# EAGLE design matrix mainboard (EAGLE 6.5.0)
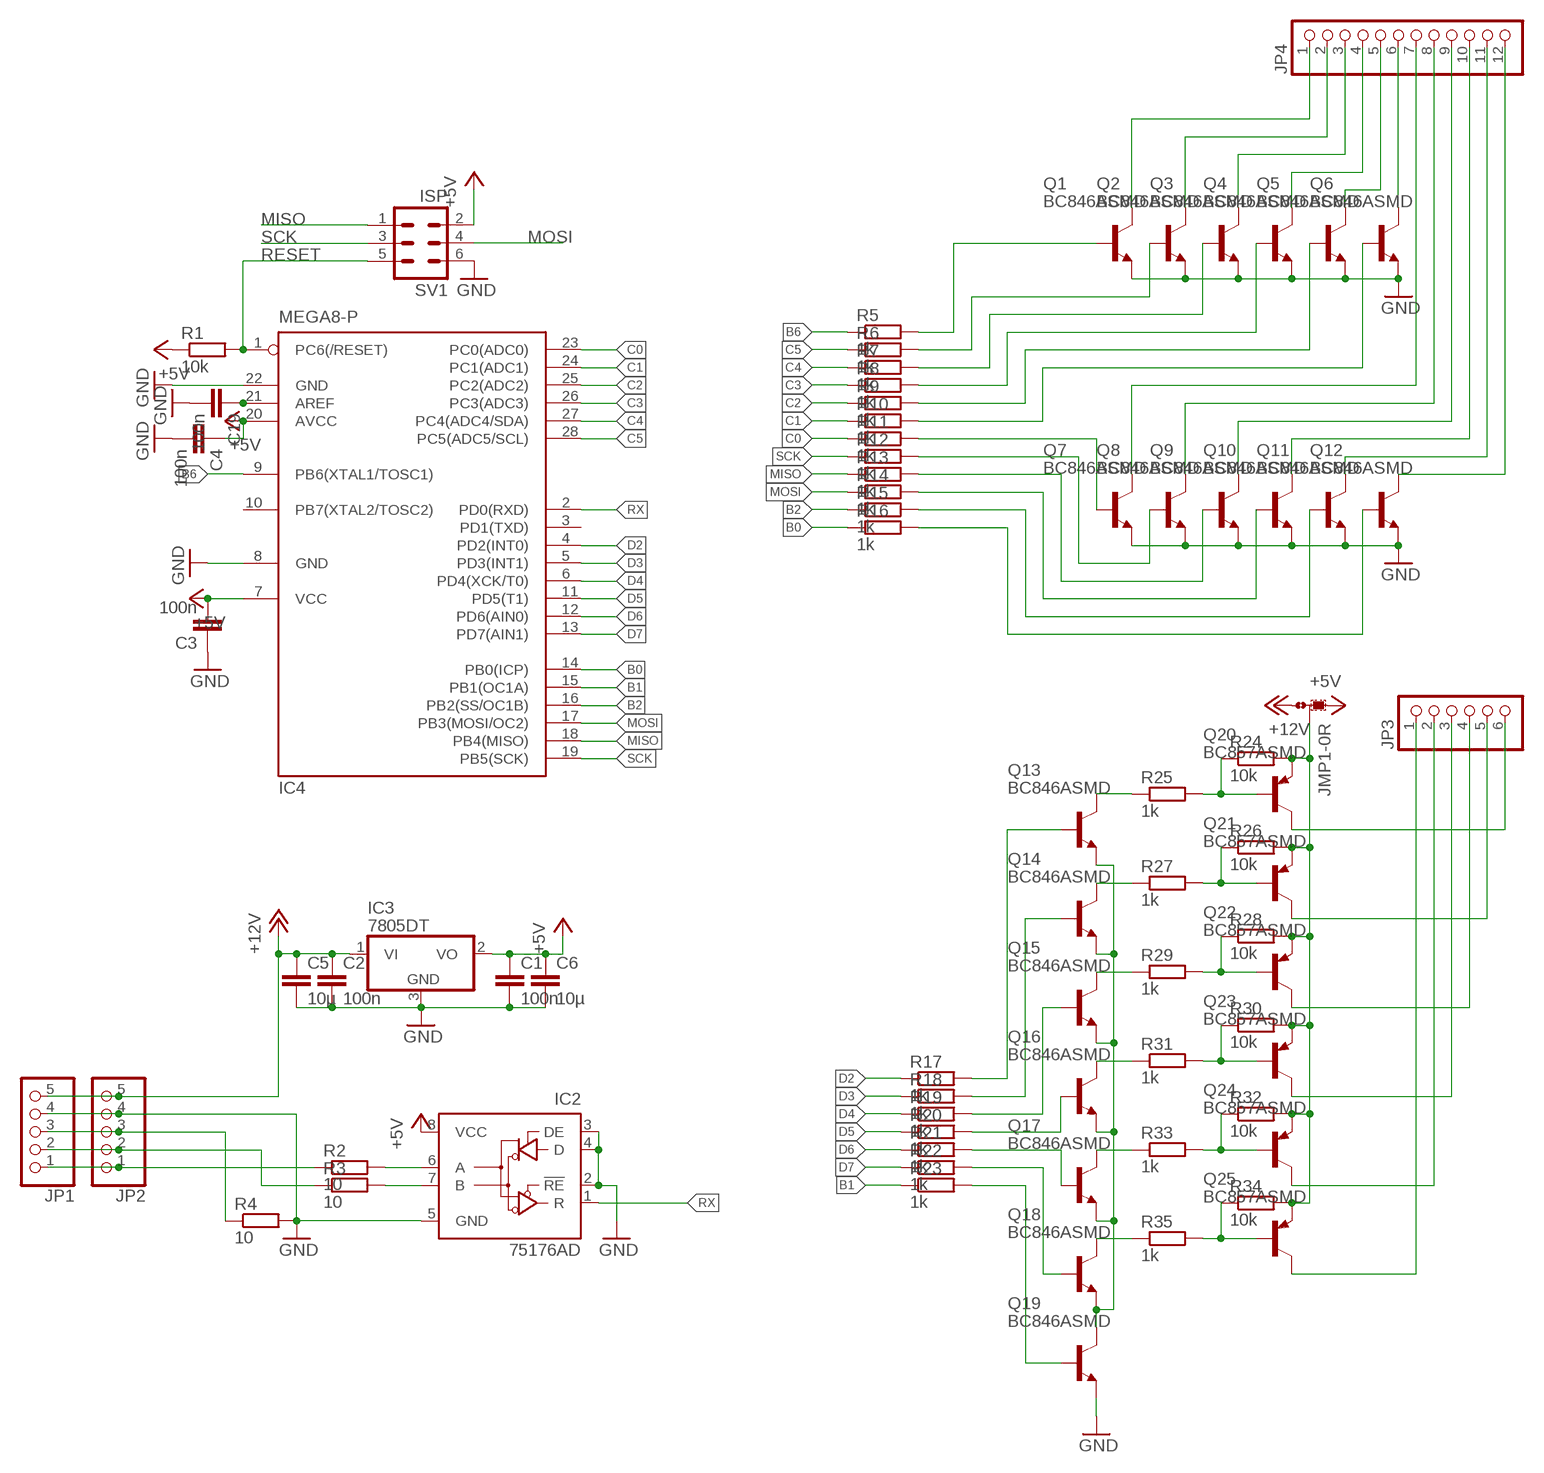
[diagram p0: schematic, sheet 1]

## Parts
C1  100n  C-EUC0805K  [C0805K]
C2  100n  C-EUC0805K  [C0805K]
C3  100n  C-EUC0805K  [C0805K]
C4  100n  C-EUC0805K  [C0805K]
C5  10µ  C-EUC0805K  [C0805K]
C6  10µ  C-EUC0805K  [C0805K]
C19  100n  C-EUC0805K  [C0805K]
IC2  75176AD  [D_R-PDSO-G8]
IC3  7805DT  [TO252]
IC4  MEGA8-P  [DIL28-3]
JMP1  0R-JUMPA  [A0R-JMP]
JP1  PINHD-1X5  [1X05]
JP2  PINHD-1X5  [1X05]
JP3  PINHD-1X6  [1X06]
JP4  PINHD-1X12  [1X12]
Q1  BC846ASMD  [SOT23]
Q2  BC846ASMD  [SOT23]
Q3  BC846ASMD  [SOT23]
Q4  BC846ASMD  [SOT23]
Q5  BC846ASMD  [SOT23]
Q6  BC846ASMD  [SOT23]
Q7  BC846ASMD  [SOT23]
Q8  BC846ASMD  [SOT23]
Q9  BC846ASMD  [SOT23]
Q10  BC846ASMD  [SOT23]
Q11  BC846ASMD  [SOT23]
Q12  BC846ASMD  [SOT23]
Q13  BC846ASMD  [SOT23]
Q14  BC846ASMD  [SOT23]
Q15  BC846ASMD  [SOT23]
Q16  BC846ASMD  [SOT23]
Q17  BC846ASMD  [SOT23]
Q18  BC846ASMD  [SOT23]
Q19  BC846ASMD  [SOT23]
Q20  BC857ASMD  [SOT23-BEC]
Q21  BC857ASMD  [SOT23-BEC]
Q22  BC857ASMD  [SOT23-BEC]
Q23  BC857ASMD  [SOT23-BEC]
Q24  BC857ASMD  [SOT23-BEC]
Q25  BC857ASMD  [SOT23-BEC]
R1  10k  R-EU_M0805  [M0805]
R2  10  R-EU_M0805  [M0805]
R3  10  R-EU_M0805  [M0805]
R4  10  R-EU_M0805  [M0805]
R5  1k  R-EU_M0805  [M0805]
R6  1k  R-EU_M0805  [M0805]
R7  1k  R-EU_M0805  [M0805]
R8  1k  R-EU_M0805  [M0805]
R9  1k  R-EU_M0805  [M0805]
R10  1k  R-EU_M0805  [M0805]
R11  1k  R-EU_M0805  [M0805]
R12  1k  R-EU_M0805  [M0805]
R13  1k  R-EU_M0805  [M0805]
R14  1k  R-EU_M0805  [M0805]
R15  1k  R-EU_M0805  [M0805]
R16  1k  R-EU_M0805  [M0805]
R17  1k  R-EU_M0805  [M0805]
R18  1k  R-EU_M0805  [M0805]
R19  1k  R-EU_M0805  [M0805]
R20  1k  R-EU_M0805  [M0805]
R21  1k  R-EU_M0805  [M0805]
R22  1k  R-EU_M0805  [M0805]
R23  1k  R-EU_M0805  [M0805]
R24  10k  R-EU_M0805  [M0805]
R25  1k  R-EU_M0805  [M0805]
R26  10k  R-EU_M0805  [M0805]
R27  1k  R-EU_M0805  [M0805]
R28  10k  R-EU_M0805  [M0805]
R29  1k  R-EU_M0805  [M0805]
R30  10k  R-EU_M0805  [M0805]
R31  1k  R-EU_M0805  [M0805]
R32  10k  R-EU_M0805  [M0805]
R33  1k  R-EU_M0805  [M0805]
R34  10k  R-EU_M0805  [M0805]
R35  1k  R-EU_M0805  [M0805]
SV1  ISP  ML6  [ML6]

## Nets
+5V: C1.1 C3.2 C4.1 C6.1 IC2.8(VCC) IC3.2(VO) IC4.7(VCC) IC4.20(AVCC) JMP1.1 R1.1 SV1.2
+12V: C2.1 C5.1 IC3.1(VI) JMP1.3 JP1.5 JP2.5
B0: IC4.14(PB0(ICP)) R16.1
B1: IC4.15(PB1(OC1A)) R23.1
B2: IC4.16(PB2(SS/OC1B)) R15.1
B6: IC4.9(PB6(XTAL1/TOSC1)) R5.1
C0: IC4.23(PC0(ADC0)) R11.1
C1: IC4.24(PC1(ADC1)) R10.1
C2: IC4.25(PC2(ADC2)) R9.1
C3: IC4.26(PC3(ADC3)) R8.1
C4: IC4.27(PC4(ADC4/SDA)) R7.1
C5: IC4.28(PC5(ADC5/SCL)) R6.1
D2: IC4.4(PD2(INT0)) R17.1
D3: IC4.5(PD3(INT1)) R18.1
D4: IC4.6(PD4(XCK/T0)) R19.1
D5: IC4.11(PD5(T1)) R20.1
D6: IC4.12(PD6(AIN0)) R21.1
D7: IC4.13(PD7(AIN1)) R22.1
GND: C1.2 C2.2 C3.1 C4.2 C5.2 C6.2 C19.2 IC2.2(!RE) IC2.3(DE) IC2.4(D) IC2.5(GND) IC3.3(GND) IC4.8(GND) IC4.22(GND) JP1.4 JP2.4 Q1.2(E) Q2.2(E) Q3.2(E) Q4.2(E) Q5.2(E) Q6.2(E) Q7.2(E) Q8.2(E) Q9.2(E) Q10.2(E) Q11.2(E) Q12.2(E) Q19.2(E) R4.2 SV1.6
MISO: IC4.18(PB4(MISO)) R13.1 SV1.1
MOSI: IC4.17(PB3(MOSI/OC2)) R14.1 SV1.4
N$1: JP1.1 JP2.1 R2.1
N$2: JP1.2 JP2.2 R3.1
N$3: JP1.3 JP2.3 R4.1
N$4: Q1.1(B) R5.2
N$6: IC2.6(A) R2.2
N$7: IC2.7(B) R3.2
N$8: Q2.1(B) R6.2
N$9: Q13.1(B) R17.2
N$10: Q14.1(B) R18.2
N$11: Q3.1(B) R7.2
N$12: Q4.1(B) R8.2
N$13: Q5.1(B) R9.2
N$14: Q6.1(B) R10.2
N$15: JP4.6 Q6.3(C)
N$16: JP4.5 Q5.3(C)
N$17: JP4.4 Q4.3(C)
N$18: JP4.3 Q3.3(C)
N$19: JP4.2 Q2.3(C)
N$20: JP4.1 Q1.3(C)
N$21: JP4.7 Q7.3(C)
N$22: JP4.8 Q8.3(C)
N$23: JP4.9 Q9.3(C)
N$24: JP4.10 Q10.3(C)
N$25: JP4.11 Q11.3(C)
N$26: JP4.12 Q12.3(C)
N$27: Q7.1(B) R11.2
N$28: Q8.1(B) R12.2
N$29: C19.1 IC4.21(AREF)
N$30: Q9.1(B) R13.2
N$31: Q10.1(B) R14.2
N$32: Q11.1(B) R15.2
N$33: Q12.1(B) R16.2
N$34: Q15.1(B) R19.2
N$35: Q16.1(B) R20.2
N$36: Q17.1(B) R21.2
N$37: Q18.1(B) R22.2
N$38: JMP1.2 Q20.E Q21.E Q22.E Q23.E Q24.E Q25.E R24.2 R26.2 R28.2 R30.2 R32.2 R34.2
N$39: Q21.B R26.1 R27.2
N$40: Q13.2(E) Q14.2(E) Q15.2(E) Q16.2(E) Q17.2(E) Q18.2(E) Q19.3(C)
N$41: Q19.1(B) R23.2
N$43: Q22.B R28.1 R29.2
N$44: Q23.B R30.1 R31.2
N$51: Q24.B R32.1 R33.2
N$52: Q25.B R34.1 R35.2
N$53: Q20.B R24.1 R25.2
N$54: Q13.3(C) R25.1
N$55: Q14.3(C) R27.1
N$56: Q15.3(C) R29.1
N$57: Q16.3(C) R31.1
N$58: Q17.3(C) R33.1
N$59: Q18.3(C) R35.1
N$60: JP3.6 Q20.C
N$61: JP3.5 Q21.C
N$62: JP3.4 Q22.C
N$63: JP3.3 Q23.C
N$64: JP3.2 Q24.C
N$65: JP3.1 Q25.C
RESET: IC4.1(PC6(/RESET)) R1.2 SV1.5
RX: IC2.1(R) IC4.2(PD0(RXD))
SCK: IC4.19(PB5(SCK)) R12.1 SV1.3
Unconnected: IC4.3(PD1(TXD)) IC4.10(PB7(XTAL2/TOSC2))

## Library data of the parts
C1-C6 C19 = rcl:C-EU: CAPACITOR, European symbol
IC2 = 751xx:75176A: DIFFERENTIAL BUS TRANSCEIVER Source: http://focus.ti.com/lit/ds/symlink/sn75176a.pdf
IC3 = linear:78*: Positive VOLTAGE REGULATOR Source: http://cache.national.com/ds/LM/LM78L05.pdf http://www.fairchildsemi.com/ds/LM/LM7805.pdf
IC4 = atmel:MEGA8-P: MICROCONTROLLER 8 Kbytes FLASH, 1 kbytes SRAM, 512 bytes EEPROM, USART, 4-channel 10 bit ADC, 2-channel 8 bit ADC Pin compatible with Atmega48, ATMega88, ATMega168 Source: avr.lbr; OC_FARNELL: unknown; OC_NEWARK: unknown
JMP1 = jump-0r-smd:0R-JUMP: SMD 0R 0805 Jumper
JP1 JP2 = pinhead:PINHD-1X5: PIN HEADER
JP3 = pinhead:PINHD-1X6: PIN HEADER
JP4 = pinhead:PINHD-1X12: PIN HEADER
Q1-Q19 = transistor-npn:BC846*: NPN Transistor
Q20-Q25 = transistor-pnp:BC857*: PNP Transistror
R1-R35 = rcl:R-EU_: RESISTOR, European symbol
SV1 = con-harting-ml:ML6: HARTING

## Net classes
0 default: width 0.4 mm, drill 0.001 mm, clearance 0.25 mm

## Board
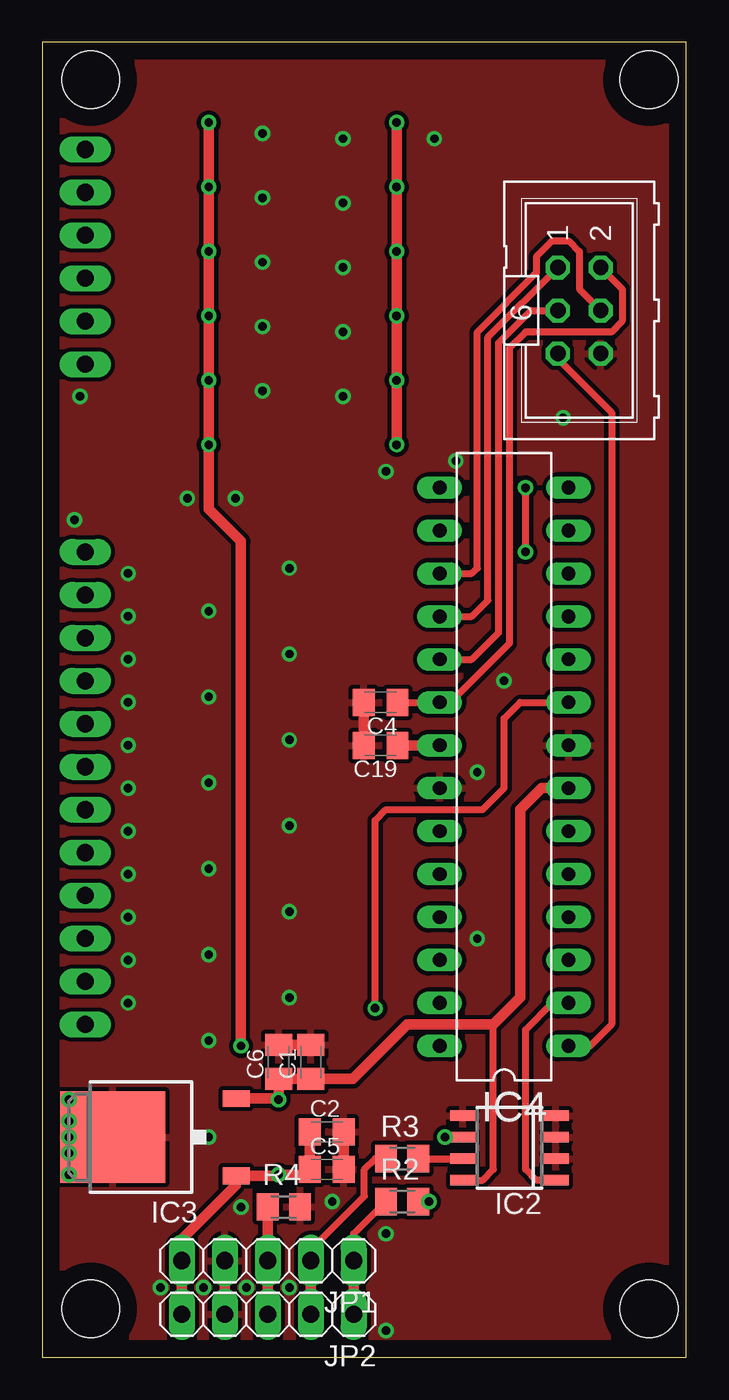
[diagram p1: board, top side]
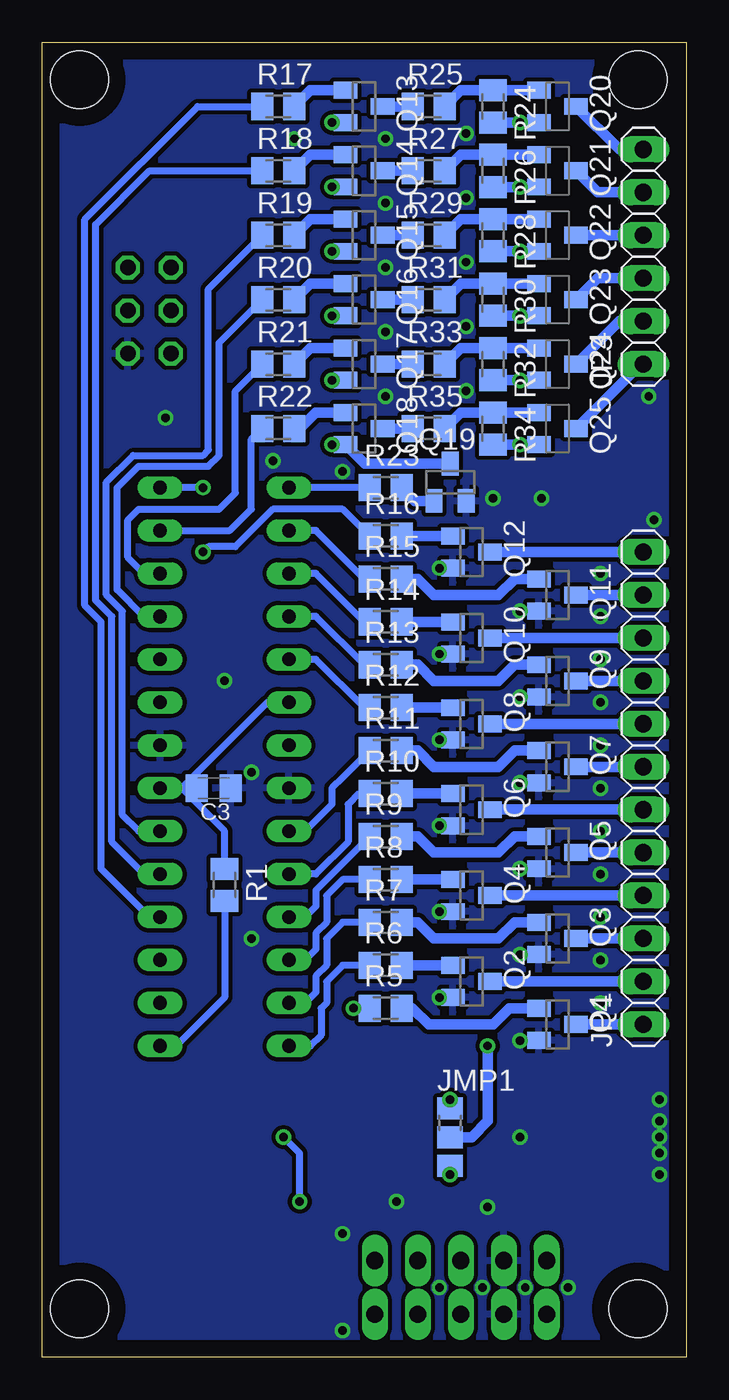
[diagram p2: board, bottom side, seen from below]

Size 38.08 x 77.78 mm. Coordinates in mm from the lower left corner, seen from the top.
Outline: 0,0 38.08,0 38.08,77.78 0,77.78 0,0
Copper layers (1*16): Top 0.035mm / dielectric 1.5mm / Bottom 0.035mm
Design rules "default": minimum track width 10mil, minimum drill 24mil, track to track 8mil, track to pad 8mil, pad to pad 8mil, via to via 8mil, smd to smd 8mil, copper to edge 40mil, drill to drill 8mil, minimum pad ring 10mil, minimum via ring 8mil, stop-mask expansion 4mil, vias tented up to drill 0mil, thermal gap 10mil
Holes 3.4 mm at 2.86,75.56 35.88,75.56 35.88,2.86 2.86,2.86

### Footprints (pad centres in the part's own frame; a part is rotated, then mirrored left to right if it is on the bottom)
C0805K = smd 1.3 x 1.6: 1 -1,0; 2 1,0
D_R-PDSO-G8 = smd 0.6 x 1.5: 1 -1.905,-2.75; 2 -0.635,-2.75; 3 0.635,-2.75; 4 1.905,-2.75; 5 1.905,2.75; 6 0.635,2.75; 7 -0.635,2.75; 8 -1.905,2.75
TO252 = smd 1 x 1.6: 1 -2.28,-4.8; 2 2.28,-4.8 | smd 5.4 x 6.2: 3 0,2.5
DIL28-3 = drill 0.813 long: 1 -16.51,-3.81; 2 -13.97,-3.81; 3 -11.43,-3.81; 4 -8.89,-3.81; 5 -6.35,-3.81; 6 -3.81,-3.81; 7 -1.27,-3.81; 8 1.27,-3.81; 9 3.81,-3.81; 10 6.35,-3.81; 11 8.89,-3.81; 12 11.43,-3.81; 13 13.97,-3.81; 14 16.51,-3.81; 15 16.51,3.81; 16 13.97,3.81; 17 11.43,3.81; 18 8.89,3.81; 19 6.35,3.81; 20 3.81,3.81; 21 1.27,3.81; 22 -1.27,3.81; 23 -3.81,3.81; 24 -6.35,3.81; 25 -8.89,3.81; 26 -11.43,3.81; 27 -13.97,3.81; 28 -16.51,3.81
A0R-JMP = smd 1.5 x 1.3: 1 0,1.7; 2 0,0; 3 0,-1.7
1X05 = drill 1.016 long: 1 -5.08,0; 2 -2.54,0; 3 0,0; 4 2.54,0; 5 5.08,0
1X06 = drill 1.016 long: 1 -6.35,0; 2 -3.81,0; 3 -1.27,0; 4 1.27,0; 5 3.81,0; 6 6.35,0
1X12 = drill 1.016 long: 1 -13.97,0; 2 -11.43,0; 3 -8.89,0; 4 -6.35,0; 5 -3.81,0; 6 -1.27,0; 7 1.27,0; 8 3.81,0; 9 6.35,0; 10 8.89,0; 11 11.43,0; 12 13.97,0
SOT23 = smd 1 x 1.4: 1 -0.95,-1.1; 2 0.95,-1.1; 3 0,1.1
SOT23-BEC = smd 1 x 1.4: B -0.95,-1.1; C 0,1.1; E 0.95,-1.1
M0805 = smd 1.3 x 1.6: 1 -0.95,0; 2 0.95,0
ML6 = drill 0.914 octagon: 1 -2.54,-1.27; 2 -2.54,1.27; 3 0,-1.27; 4 0,1.27; 5 2.54,-1.27; 6 2.54,1.27

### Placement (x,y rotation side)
C1  15.88,17.46 90 top
C2  16.83,13.33 0 top
C3  27.94,33.65 180 bottom
C4  20,38.73 180 top
C5  16.83,11.11 0 top
C6  13.97,17.46 90 top
C19  20,36.2 180 top
IC2  27.62,12.38 90 top
IC3  6.67,13.02 90 top
IC4  27.3,34.92 90 top
JMP1  13.97,13.02 0 bottom
JP1  13.34,5.71 180 top
JP2  13.34,2.54 180 top
JP3  2.54,65.09 90 bottom
JP4  2.54,33.65 90 bottom
Q1  7.62,19.69 270 bottom
Q2  12.7,22.23 270 bottom
Q3  7.62,24.77 270 bottom
Q4  12.7,27.3 270 bottom
Q5  7.62,29.85 270 bottom
Q6  12.7,32.38 270 bottom
Q7  7.62,34.92 270 bottom
Q8  12.7,37.46 270 bottom
Q9  7.62,40 270 bottom
Q10  12.7,42.54 270 bottom
Q11  7.62,45.09 270 bottom
Q12  12.7,47.62 270 bottom
Q13  19.05,73.98 270 bottom
Q14  19.05,70.17 270 bottom
Q15  19.05,66.36 270 bottom
Q16  19.05,62.55 270 bottom
Q17  19.05,58.74 270 bottom
Q18  19.05,54.93 270 bottom
Q19  13.97,51.75 0 bottom
Q20  7.62,73.98 270 bottom
Q21  7.62,70.17 270 bottom
Q22  7.62,66.36 270 bottom
Q23  7.62,62.55 270 bottom
Q24  7.62,58.74 270 bottom
Q25  7.62,54.93 270 bottom
R1  27.3,27.94 270 bottom
R2  21.27,9.21 0 top
R3  21.27,11.75 0 top
R4  14.29,8.89 0 top
R5  17.78,20.64 0 bottom
R6  17.78,23.18 0 bottom
R7  17.78,25.72 0 bottom
R8  17.78,28.26 0 bottom
R9  17.78,30.8 0 bottom
R10  17.78,33.34 0 bottom
R11  17.78,35.88 0 bottom
R12  17.78,38.42 0 bottom
R13  17.78,40.96 0 bottom
R14  17.78,43.5 0 bottom
R15  17.78,46.04 0 bottom
R16  17.78,48.58 0 bottom
R17  24.13,73.98 0 bottom
R18  24.13,70.17 0 bottom
R19  24.13,66.36 0 bottom
R20  24.13,62.55 0 bottom
R21  24.13,58.74 0 bottom
R22  24.13,54.93 0 bottom
R23  17.78,51.43 0 bottom
R24  11.43,73.98 270 bottom
R25  15.24,73.98 0 bottom
R26  11.43,70.17 270 bottom
R27  15.24,70.17 0 bottom
R28  11.43,66.36 270 bottom
R29  15.24,66.36 0 bottom
R30  11.43,62.55 270 bottom
R31  15.24,62.55 0 bottom
R32  11.43,58.74 270 bottom
R33  15.24,58.74 0 bottom
R34  11.43,54.93 270 bottom
R35  15.24,54.93 0 bottom
SV1  31.75,61.91 270 top

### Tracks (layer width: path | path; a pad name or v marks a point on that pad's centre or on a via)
+5V  (via drill 0.5)
  Top 0.406: C4.1 IC4.20 24.13,38.74 27.62,42.23 27.62,59.69 28.57,60.64 33.66,60.64 34.29,61.28 34.29,63.18 SV1.2 | IC2.8 26.04,10.48 26.67,11.11 26.67,19.69
  Top 0.61: IC4.7 29.53,33.65 28.26,32.39 28.26,21.27 26.67,19.69 21.59,19.69 18.37,16.46 C6.1 | C1.1 C6.1 | IC3.2 13.91,15.3 v13.97,15.24 C6.1
  Bottom 0.406: R1.1 27.3,31.12 29.84,33.65 | 29.84,33.65 IC4.7 | 29.84,33.65 24.77,38.74 IC4.20 | C3.2 29.84,33.65
  Bottom 0.61: v13.97,15.24 13.97,14.92 13.87,14.82 JMP1.1
+12V  (via drill 0.5)
  Top 0.61: JP2.5 JP1.5 8.26,6.99 11.43,10.16 11.43,10.7 IC3.1 13.91,10.74 v13.97,10.8 15.56,10.8 15.83,11.07 C2.1 C5.1
  Bottom 0.61: v13.97,10.8 JMP1.3
B0  (via drill 0.5)
  Top 0.406: v28.57,47.63 v28.57,51.43
  Bottom 0.406: v28.57,47.63 28.26,47.94 26.67,47.94 24.45,50.17 20.32,50.17 R16.1 | v28.57,51.43 IC4.14
B1
  Bottom 0.406: R23.1 IC4.15
B2
  Bottom 0.406: R15.1 19.05,46.04 21.91,48.89 IC4.16
B6  (via drill 0.5)
  Top 0.406: v19.68,20.64 19.68,31.75 20.32,32.39 26.04,32.39 27.3,33.65 27.3,37.78 28.26,38.74 IC4.9
  Bottom 0.406: R5.1 v19.68,20.64
C0
  Bottom 0.406: R11.1 20.32,34.29 20.95,33.65 20.95,32.7 22.54,31.12 IC4.23
C1
  Bottom 0.406: R10.1 19.37,33.34 20,32.7 20,30.48 21.91,28.57 IC4.24
C2
  Bottom 0.406: R9.1 21.91,27.62 21.91,26.67 22.54,26.03 IC4.25
C3
  Bottom 0.406: IC4.26 22.54,23.49 21.91,24.13 21.91,25.08 21.27,25.72 21.27,27.3 20.32,28.26 R8.1
C4
  Bottom 0.406: IC4.27 22.54,20.96 21.91,21.59 21.91,22.54 21.27,23.18 21.27,24.76 20.32,25.72 R7.1
C5
  Bottom 0.406: IC4.28 22.23,18.42 21.59,19.05 21.59,20.64 21.27,20.96 21.27,22.23 20.32,23.18 R6.1
D2
  Bottom 0.406: IC4.4 31.75,26.03 34.61,28.89 34.61,43.5 35.56,44.45 35.56,67.31 28.89,73.98 R17.1
D3
  Bottom 0.406: IC4.5 32.07,28.57 33.97,30.48 33.97,43.82 34.92,44.77 34.92,66.99 31.75,70.17 R18.1
D4
  Bottom 0.406: IC4.6 32.38,31.12 33.34,32.07 33.34,44.13 34.29,45.09 34.29,51.75 32.7,53.34 28.57,53.34 28.26,53.66 28.26,63.18 R19.1
D5
  Bottom 0.406: IC4.11 32.07,43.82 33.66,45.4 33.66,51.43 32.38,52.71 28.26,52.71 27.62,53.34 27.62,60 R20.1
D6
  Bottom 0.406: IC4.12 32.07,46.35 33.02,47.31 33.02,49.53 32.38,50.17 27.62,50.17 26.67,51.12 26.67,57.15 R21.1
D7
  Bottom 0.406: IC4.13 26.99,48.89 25.72,50.17 25.72,54.29 R22.1
GND  (via drill 0.5)
  Top 0.61: JP2.4 JP1.4 | C19.2 C4.2 | C5.2 C2.2 | C1.2 C6.2
  other vias: 14.61,21.27 14.61,26.35 14.61,31.43 14.61,36.51 14.61,41.59 14.61,46.67 11.43,50.8 8.57,50.8 23.18,72.07 17.78,56.83 17.78,60.64 17.78,64.45 17.78,72.07 13.02,57.15 13.02,60.96 13.02,64.77 13.02,68.58 13.02,72.39 24.45,53.02 20.32,52.39 30.8,55.56 17.78,68.26 1.59,10.79 1.59,12.06 1.59,13.02 1.59,13.97 1.59,15.24 25.72,24.77 27.3,40 25.72,34.61 9.84,28.89 9.84,23.81 9.84,18.73 9.84,33.97 9.84,39.05 9.84,44.13 5.08,46.35 5.08,43.81 5.08,41.27 5.08,38.73 5.08,36.2 5.08,33.65 5.08,31.12 5.08,28.57 5.08,26.04 5.08,23.5 5.08,20.96 2.22,56.83 1.91,49.53 11.75,8.89 17.14,9.21 20.32,7.3 20.32,1.59 14.61,4.13 12.06,4.13 9.53,4.13 6.99,4.13 9.84,13.02
  pour Bottom: 0.32,0 0.32,77.47 37.78,77.47 37.78,0
  pour Top: 0.32,0 0.32,77.47 37.78,77.47 37.78,0
MISO
  Top 0.406: IC4.18 25.4,43.82 26.35,44.77 26.35,60.32 SV1.1
  Bottom 0.406: R13.1 19.05,40.96 21.91,43.82 IC4.18
MOSI
  Top 0.406: IC4.17 25.4,46.35 25.72,46.67 25.72,60.64 29.21,64.14 29.21,65.09 30.16,66.04 31.11,66.04 31.75,65.4 31.75,63.18 SV1.4
  Bottom 0.406: R14.1 19.05,43.5 21.91,46.35 IC4.17
N$1
  Top 0.406: JP1.1 18.41,7.3 R2.1
  Top 0.61: JP2.1 JP1.1
N$2
  Top 0.406: JP1.2 15.88,6.35 19.05,9.52 19.05,11.11 19.68,11.75 R3.1
  Top 0.61: JP2.2 JP1.2
N$3
  Top 0.61: JP2.3 JP1.3 R4.1
N$4
  Bottom 0.61: R5.2 16.19,20.64 15.24,19.69 11.43,19.69 10.48,20.64 Q1.1
N$6  (via drill 0.5)
  Top 0.406: R2.2 v22.86,9.21 | v23.81,13.02 IC2.6
  Bottom 0.406: v22.86,9.21 22.86,12.07 v23.81,13.02
N$7
  Top 0.406: R3.2 IC2.7
N$8
  Bottom 0.61: R6.2 Q2.1
N$9
  Bottom 0.61: R17.2 22.23,74.93 Q13.1
N$10
  Bottom 0.61: R18.2 22.23,71.12 Q14.1
N$11
  Bottom 0.61: R7.2 15.88,25.72 14.92,24.76 11.11,24.76 10.16,25.72 Q3.1
N$12
  Bottom 0.61: R8.2 Q4.1
N$13
  Bottom 0.61: R9.2 15.88,30.8 14.92,29.85 11.11,29.85 10.16,30.8 Q5.1
N$14
  Bottom 0.61: R10.2 Q6.1
N$15
  Bottom 0.61: Q6.3 JP4.6
N$16
  Bottom 0.61: Q5.3 JP4.5
N$17
  Bottom 0.61: Q4.3 JP4.4
N$18
  Bottom 0.61: Q3.3 JP4.3
N$19
  Bottom 0.61: Q2.3 JP4.2
N$20
  Bottom 0.61: JP4.1 Q1.3
N$21
  Bottom 0.61: Q7.3 JP4.7
N$22
  Bottom 0.61: Q8.3 JP4.8
N$23
  Bottom 0.61: Q9.3 JP4.9
N$24
  Bottom 0.61: Q10.3 JP4.10
N$25
  Bottom 0.61: Q11.3 JP4.11
N$26
  Bottom 0.61: Q12.3 JP4.12
N$27
  Bottom 0.61: R11.2 15.88,35.88 14.92,34.92 11.11,34.92 10.16,35.88 Q7.1
N$28
  Bottom 0.61: R12.2 Q8.1
N$29
  Top 0.61: C19.1 IC4.21
N$30
  Bottom 0.61: R13.2 15.88,40.96 14.92,40 11.11,40 10.16,40.96 Q9.1
N$31
  Bottom 0.61: R14.2 Q10.1
N$32
  Bottom 0.61: R15.2 15.88,46.04 14.92,45.09 11.11,45.09 10.16,46.04 Q11.1
N$33
  Bottom 0.61: R16.2 Q12.1
N$34
  Bottom 0.61: R19.2 22.23,67.31 Q15.1
N$35
  Bottom 0.61: R20.2 22.23,63.5 Q16.1
N$36
  Bottom 0.61: R21.2 22.23,59.69 Q17.1
N$37
  Bottom 0.61: R22.2 22.86,54.93 21.91,55.88 Q18.1
N$38  (via drill 0.5)
  Top 0.61: v9.84,73.03 v9.84,69.22 | v9.84,69.22 v9.84,65.4 v9.84,61.6 v9.84,57.78 v9.84,53.98 9.84,50.17 11.75,48.26 v11.75,18.42 | v9.84,69.22 v9.85,69.22 v9.84,69.21
  Bottom 0.61: R30.2 Q23.E v9.84,61.6 | R32.2 Q24.E v9.84,57.79 v9.84,57.78 | R34.2 v9.84,53.98 Q25.E | R28.2 Q22.E v9.84,65.41 v9.84,65.4 | R26.2 v9.84,69.21 | R24.2 Q20.E v9.84,73.03 | Q21.E v9.84,69.21 | v9.84,69.21 | JMP1.2 12.7,13.02 11.75,13.97 v11.75,18.42
N$39
  Bottom 0.61: Q21.B R26.1 13.34,71.12 R27.2
N$40  (via drill 0.5)
  Top 0.61: v20.95,73.03 v20.95,69.21 v20.95,65.4 v20.95,61.6 v20.95,57.78 v20.95,53.97
  Bottom 0.61: Q19.3 19.02,52.85 Q18.2 v20.95,53.97 | Q13.2 v20.95,73.03 | Q17.2 v20.95,57.79 v20.95,57.78 | Q16.2 v20.95,61.6 | Q15.2 v20.95,65.41 v20.95,65.4 | Q14.2 v20.95,69.22 v20.95,69.21
N$41
  Bottom 0.61: Q19.1 16.05,50.65 R23.2
N$43
  Bottom 0.61: Q22.B R28.1 13.34,67.31 R29.2
N$44
  Bottom 0.61: R31.2 13.34,63.5 R30.1 Q23.B
N$51
  Bottom 0.61: R33.2 13.34,59.69 R32.1 Q24.B
N$52
  Bottom 0.61: R35.2 13.34,55.88 R34.1 Q25.B
N$53
  Bottom 0.61: Q20.B R24.1 13.34,74.93 R25.2
N$54
  Bottom 0.61: Q13.3 R25.1
N$55
  Bottom 0.61: Q14.3 R27.1
N$56
  Bottom 0.61: Q15.3 R29.1
N$57
  Bottom 0.61: Q16.3 R31.1
N$58
  Bottom 0.61: Q17.3 R33.1
N$59
  Bottom 0.61: Q18.3 R35.1
N$60
  Bottom 0.61: JP3.6 3.98,71.44 Q20.C
N$61
  Bottom 0.61: JP3.5 5.25,68.9 Q21.C
N$62
  Bottom 0.61: JP3.4 Q22.C
N$63
  Bottom 0.61: JP3.3 5.25,63.82 Q23.C
N$64
  Bottom 0.61: JP3.2 3.98,61.28 Q24.C
N$65
  Bottom 0.61: JP3.1 2.71,58.74 Q25.C
RESET
  Top 0.406: SV1.5 30.48,59.06 33.66,55.88 33.66,19.69 32.38,18.42 IC4.1
  Bottom 0.406: R1.2 27.3,21.27 30.16,18.42 IC4.1
RX
  Top 0.406: IC2.1 29.21,10.48 28.57,11.11 28.57,19.37 30.16,20.96 IC4.2
SCK
  Top 0.406: IC4.19 25.4,41.28 26.99,42.86 26.99,60.01 28.89,61.91 SV1.3
  Bottom 0.406: R12.1 19.05,38.42 21.91,41.28 IC4.19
